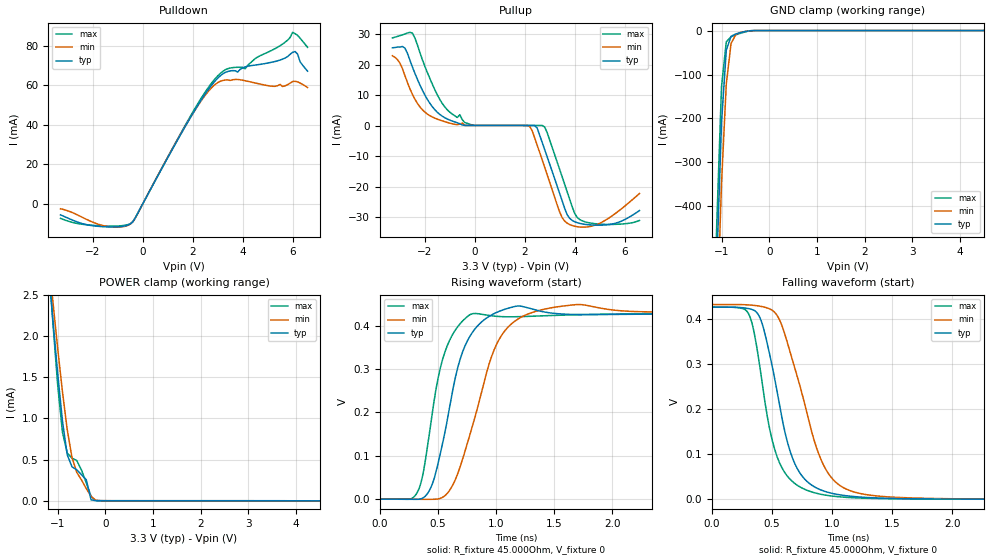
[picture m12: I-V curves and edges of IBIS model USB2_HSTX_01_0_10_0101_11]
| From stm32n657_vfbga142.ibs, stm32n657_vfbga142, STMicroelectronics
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[Model] USB2_HSTX_01_0_10_0101_11
Model_type   Output
Polarity   Non-Inverting
Enable   Active-High
C_comp   8.036pF   7.631pF   8.569pF
Vmeas = 200.000mV
Vref = 200.000mV
Rref = 45Ohms
Cref = 0pF
[Model Spec]
Vmeas   200.000mV   200.000mV   200.000mV
Vref   200.000mV   200.000mV   200.000mV
| This model is not intended for timing simulations.
| Warnings about Cref, Vref & Rref can be ignored
[Temperature Range]   25.000   125.000   -40.000
[Voltage Range]   3.300V   3.070V   3.630V
[GND Clamp Reference]   0.00V   0.00V   0.00V
[Pulldown Reference]   0.00V   0.00V   0.00V
[POWER Clamp Reference]   3.300V   3.070V   3.630V
[Pullup Reference]   3.300V   3.070V   3.630V
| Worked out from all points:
|   slope of the pulldown table from 0 to 0.495 V, typ, clamps not added: 42.6 ohm
|   GND clamp passes 1 mA (typ) near -0.43 V on its own axis
|   POWER clamp passes 1 mA (typ) near -0.91 V on its own axis
|   rising waveform, R_fixture 45.000Ohm, V_fixture 0: 20-80 % time 213ps typ, 282ps min, 175ps max; typ from 0 V to 0.428 V
|   falling waveform, R_fixture 45.000Ohm, V_fixture 0: 20-80 % time 215ps typ, 280ps min, 185ps max; typ from 0.427 V to 0 V
[GND Clamp]
-3.3V     -11.02A    -10.62A    -11.32A
-1.2V     -931.6mA   -1.049A    -855.7mA
-1.1V     -533.1mA   -671.7mA   -440.2mA
-1V       -209.4mA   -347mA     -127.3mA
-900mV    -44.44mA   -121.7mA   -25.6mA
-800mV    -13.15mA   -29.48mA   -14.15mA
-700mV    -7.742mA   -9.125mA   -9.769mA
-500mV    -2.127mA   -1.981mA   -2.894mA
-300mV    -19.47uA   -62.22uA   -13.56uA
6.6V      10.37uA    26.59uA    21.05uA
[Power Clamp]
-3.3V     3.206A     2.175A     4.855A
-1.2V     2.88mA     3.008mA    2.969mA
-1.1V     2.195mA    2.419mA    2.156mA
-1V       1.545mA    1.852mA    1.406mA
-900mV    967.5uA    1.324mA    831.4uA
-800mV    558.4uA    864.6uA    580.3uA
-700mV    412uA      525.9uA    517uA
-600mV    376.6uA    345uA      488.5uA
-400mV    254.2uA    146.6uA    216.8uA
-300mV    11.21uA    52.87uA    53.51uA
-100mV    94.86nA    984.9nA    361.1nA
6.6V      -2.721uA   -5.181uA   -3.917uA
[Pulldown]
-3.3V     -5.671mA   -2.581mA   -7.449mA
-1.6V     -11.64mA   -11.09mA   -11.31mA
-500mV    -10.25mA   -10.32mA   -10.1mA
1.9V      43.42mA    43.46mA    44.13mA
2.9V      62.15mA    60.37mA    63.26mA
3.4V      66.87mA    62.63mA    68.29mA
4.1V      69.19mA    62.19mA    68.26mA
4.5V      70.11mA    61.06mA    73.4mA
5.6V      73.12mA    59.29mA    80.76mA
6V        76.56mA    61.79mA    86.69mA
6.1V      76.96mA    61.93mA    85.99mA
6.6V      67.05mA    58.79mA    79.1mA
[Pullup]
-3.3V     25.47mA    22.87mA    28.69mA
-2.8V     25.39mA    16.38mA    30mA
-2.5V     19.21mA    10.28mA    30.27mA
-1.7V     6.185mA    2.827mA    13.54mA
-400mV    111.7uA    77.66uA    1.021mA
2.2V      68.65uA    -248.9uA   104.8uA
2.5V      -770.8uA   -6.355mA   83.48uA
2.8V      -7.785mA   -13.58mA   -409.6uA
3.4V      -22.12mA   -28.2mA    -14.26mA
3.8V      -30.28mA   -32.32mA   -24mA
4.4V      -32.24mA   -33.17mA   -31.39mA
6.6V      -27.75mA   -22.18mA   -30.98mA
[Ramp]
R_load=45.000Ohm
dV/dt_r   628.626mV/1.040ns  596.897mV/1.070ns  682.272mV/975.000ps
dV/dt_f   630.820mV/240.000ps  599.812mV/315.000ps  684.093mV/215.000ps
[Rising waveform]
R_fixture=45.000Ohm
V_fixture=0
0s        452nV      3.134uV    468nV
330ps     -314.7uV   -409.1uV   20.75mV
450ps     34.95mV    -426uV     199.2mV
590ps     198.7mV    17.05mV    361mV
680ps     314.1mV    67.14mV    401.5mV
780ps     378.2mV    154.4mV    426mV
980ps     427.4mV    342.8mV    421.9mV
1.17ns    444.7mV    412.1mV    420.4mV
1.71ns    425.4mV    448.7mV    425.2mV
9.9ns     427.9mV    433.7mV    427.8mV
[Falling waveform]
R_fixture=45.000Ohm
V_fixture=0
0s        427.4mV    433.2mV    427.3mV
310ps     423.7mV    432.1mV    409.5mV
410ps     396.3mV    428.9mV    273mV
540ps     241.5mV    409.4mV    95.78mV
620ps     134.7mV    354.7mV    53.96mV
700ps     73.04mV    281.9mV    32.99mV
950ps     16.69mV    65mV       9.102mV
1.17ns    6.449mV    17.31mV    3.528mV
1.71ns    1.126mV    2.679mV    820.1uV
9.9ns     14.1uV     31.02uV    4.407uV
